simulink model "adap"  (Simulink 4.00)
settings: Solver=ode2  SolverMode=SingleTasking  StartTime=0.0  StopTime=max(t)  RelTol=1e-2  AbsTol=1e-4
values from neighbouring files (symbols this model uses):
  h = 1/8192    (= 0.0001220703125)    [tryit.m]
libraries: simulink_extras x2

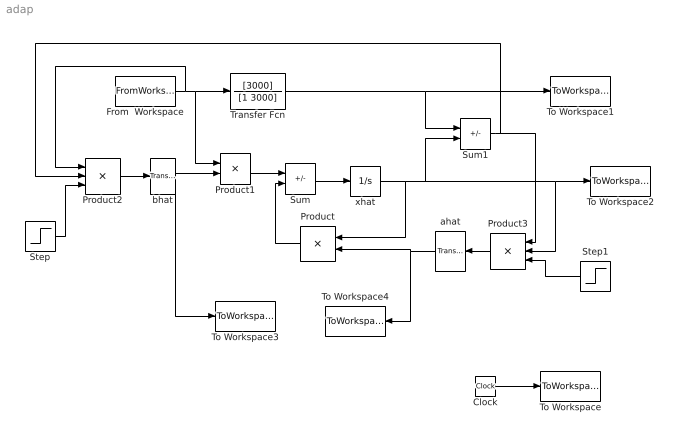
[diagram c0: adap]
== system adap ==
  Clock : Clock
  From  Workspace : FromWorkspace  VariableName=[t,u]  SampleTime=-1  OutputAfterFinalValue=Extrapolation
  Product : Product  Orientation=left  Inputs=2  Multiplication=Element-wise(.*)  SaturateOnIntegerOverflow=on
  Product1 : Product  Inputs=2  Multiplication=Element-wise(.*)  SaturateOnIntegerOverflow=on
  Product2 : Product  Inputs=3  Multiplication=Element-wise(.*)  SaturateOnIntegerOverflow=on
  Product3 : Product  Orientation=left  Inputs=3  Multiplication=Element-wise(.*)  SaturateOnIntegerOverflow=on
  Step : Step  Time=10  Before=0  After=1e5  SampleTime=h
  Step1 : Step  Orientation=left  Time=10  Before=0  After=-1e5  SampleTime=h
  Sum : Sum  Inputs=+-  SaturateOnIntegerOverflow=on
  Sum1 : Sum  Inputs=+-  SaturateOnIntegerOverflow=on
  To Workspace : ToWorkspace  VariableName=simout  SampleTime=-1  SaveFormat=Array
  To Workspace1 : ToWorkspace  VariableName=x  SampleTime=h  SaveFormat=Array
  To Workspace2 : ToWorkspace  VariableName=xhat  SampleTime=h  SaveFormat=Array
  To Workspace3 : ToWorkspace  VariableName=bhat  SampleTime=h  SaveFormat=Array
  To Workspace4 : ToWorkspace  VariableName=ahat  SampleTime=h  SaveFormat=Array
  Transfer Fcn : TransferFcn  Numerator=[3000]  Denominator=[1 3000]  Realization=auto  AbsoluteTolerance=auto
  ahat : simulink_extras/Additional Linear/Transfer Fcn (with initial states)  Orientation=left  N=[1]  D="[1  0]"  X0=0
  bhat : simulink_extras/Additional Linear/Transfer Fcn (with initial states)  N=[1]  D="[1  0]"  X0=0
  xhat : Integrator  ExternalReset=none  InitialConditionSource=internal  InitialCondition=0  LimitOutput=off  UpperSaturationLimit=inf  LowerSaturationLimit=-inf  ShowSaturationPort=off  ShowStatePort=off  AbsoluteTolerance=auto
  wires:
  Clock/1 -> To Workspace/1
  Product1/1 -> Sum/1
  Sum/1 -> xhat/1
  Product/1 -> Sum/2
  xhat/1 -> Product/1, Sum1/2, To Workspace2/1, Product3/2
  Transfer Fcn/1 -> To Workspace1/1, Sum1/1
  Product2/1 -> bhat/1
  From  Workspace/1 -> Transfer Fcn/1, Product1/1, Product2/1
  Product3/1 -> ahat/1
  Step1/1 -> Product3/3
  Sum1/1 -> Product2/2, Product3/1
  Step/1 -> Product2/3
  bhat/1 -> Product1/2, To Workspace3/1
  ahat/1 -> Product/2, To Workspace4/1
